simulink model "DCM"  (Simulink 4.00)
settings: Solver=ode45  StartTime=0.0  StopTime=10.0  RelTol=1e-3

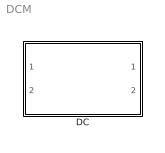
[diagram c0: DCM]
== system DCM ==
  DC : Subsystem  mask(Permanently excited DC machine){Ra=0.5, La=0.02, Psim=1.0, J=0.05, wro=0}
      mask prompts: Ra "Rotor resistance [1/2]"; La "Rotor inductance [H]"; Psim "Magnetizing flux linkage [Vs]"; J "Inertia [kgm2]"; wro "Starting speed [rad(s)]"
      mask init:
      | Ra=1

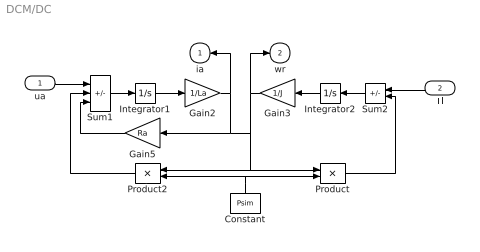
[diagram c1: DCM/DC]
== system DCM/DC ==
  ua : Inport  Port=1  LatchInput=off
  Tl : Inport  Orientation=left  Port=2  LatchInput=off
  Constant : Constant  Orientation=up  Value=Psim
  Gain2 : Gain  Gain=1/La  Multiplication=Element-wise(K.*u)  SaturateOnIntegerOverflow=on
  Gain3 : Gain  Orientation=left  Gain=1/J  Multiplication=Element-wise(K.*u)  SaturateOnIntegerOverflow=on
  Gain5 : Gain  Orientation=left  Gain=Ra  Multiplication=Element-wise(K.*u)  SaturateOnIntegerOverflow=on
  Integrator1 : Integrator  ExternalReset=none  InitialConditionSource=internal  InitialCondition=0  LimitOutput=off  UpperSaturationLimit=inf  LowerSaturationLimit=-inf  ShowSaturationPort=off  ShowStatePort=off  AbsoluteTolerance=auto
  Integrator2 : Integrator  Orientation=left  ExternalReset=none  InitialConditionSource=internal  InitialCondition=wro  LimitOutput=off  UpperSaturationLimit=inf  LowerSaturationLimit=-inf  ShowSaturationPort=off  ShowStatePort=off  AbsoluteTolerance=auto
  Product : Product  Inputs=2  Multiplication=Element-wise(.*)  SaturateOnIntegerOverflow=on
  Product2 : Product  Orientation=left  Inputs=2  Multiplication=Element-wise(.*)  SaturateOnIntegerOverflow=on
  Sum1 : Sum  Inputs=+--  SaturateOnIntegerOverflow=on
  Sum2 : Sum  Orientation=left  Inputs=-+  SaturateOnIntegerOverflow=on
  ia : Outport  Orientation=left  Port=1  InitialOutput=0
  wr : Outport  Port=2  InitialOutput=0
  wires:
  Gain5/1 -> Sum1/3
  Constant/1 -> Product2/2, Product/2
  ua/1 -> Sum1/1
  Product2/1 -> Sum1/2
  Integrator1/1 -> Gain2/1
  Tl/1 -> Sum2/1
  Product/1 -> Sum2/2
  Sum2/1 -> Integrator2/1
  Integrator2/1 -> Gain3/1
  Sum1/1 -> Integrator1/1
  Gain2/1 -> Gain5/1, Product/1, ia/1
  Gain3/1 -> Product2/1, wr/1
